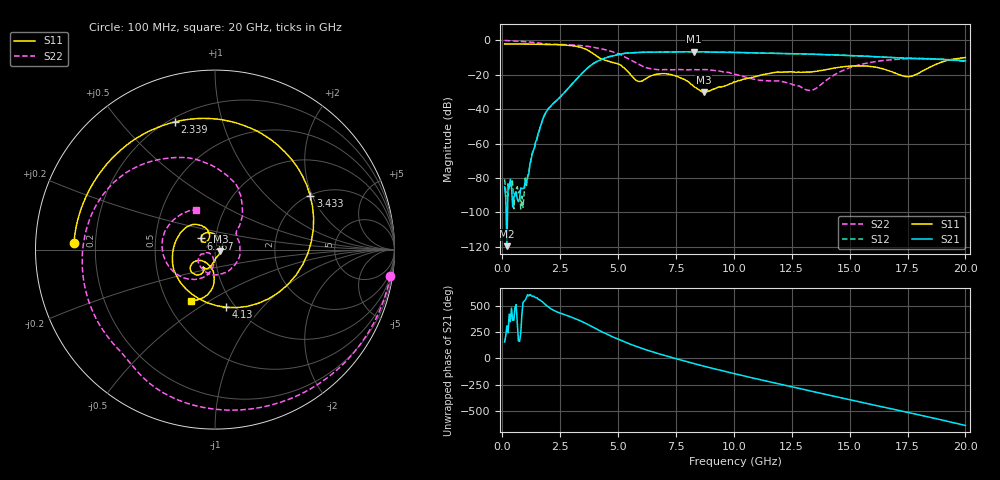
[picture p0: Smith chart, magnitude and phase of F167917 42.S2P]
!  2-Port S-parameters saved by WinCal
! VAR MeasName=S-Parameters (CALIBRATED_DATA) read from VNA (N5242A)
! VAR MeasDate=2016-11-22 9:01:51
! VAR NAME=F167917 42
! VAR FILENAME=F167917 42.S2P
! VAR DATE=2016-11-22 9:01:51
! VAR PHYS_PORTS=1,2
# Hz S DB R 50
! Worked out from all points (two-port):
!   401 points, 100 MHz to 20 GHz, reference 50 ohm
!   highest |S21| = -6.61 dB at 8.259 GHz (marker M1); lowest = -119.6 dB at 199.5 MHz (marker M2)
!   |S21| within 3 dB of the highest: 4.596 GHz to 16.25 GHz (11.66 GHz wide, 112 % of centre)
!   lowest |S11| = -30.1 dB at 8.707 GHz (marker M3), VSWR 1.06, Z = 53.1 - j0.995 ohm
!   |S11| at or under -10 dB: 4.166 GHz to end of sweep
!   |S22| runs from -29.1 to -0.1 dB; largest |S21 - S12| = 0.0059
!   S11 on the Smith chart (normalised r, x): 100 MHz: 0.12, +0.02; 2.339 GHz: 0.22, +0.71; 3.433 GHz: 2.03, +1.93; 4.13 GHz: 0.91, -0.65; 6.567 GHz: 0.85, +0.11; 20 GHz: 0.66, -0.42
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1e8  -2.09 177.3  -85.10 156.0  -80.76 154.0  -0.10 -8.7
1.995e8  -2.10 174.7  -119.60 -49.3  -90.77 -77.3  -0.16 -16.9
1.04525e9  -2.23 151.9  -82.88 -137.0  -84.39 -79.3  -0.87 -80.9
1.74175e9  -2.35 130.7  -46.18 179.4  -46.16 179.3  -1.95 -124.1
2.33875e9  -2.55 107.4  -35.04 86.1  -34.99 85.9  -2.33 -151.7
2.93575e9  -3.03 74.0  -26.60 37.7  -26.63 37.6  -2.65 -180.0
3.43325e9  -4.30 29.5  -19.34 -7.8  -19.36 -7.7  -3.10 156.1
4.12975e9  -9.70 -79.1  -12.03 -87.1  -11.99 -87.1  -4.57 121.9
4.5775e9  -12.11 -162.6  -9.67 -135.1  -9.63 -135.4  -5.95 99.8
5.22425e9  -15.66 123.7  -7.76 163.3  -7.75 163.0  -9.15 67.5
5.871e9  -23.83 127.1  -7.07 107.9  -7.07 107.8  -13.82 46.0
6.5675e9  -19.98 141.8  -6.90 57.2  -6.90 57.0  -16.77 34.8
6.7665e9  -19.51 134.3  -6.85 43.9  -6.86 43.7  -17.10 29.2
8.259e9  -26.73 37.5  -6.61 -48.1  -6.63 -48.0  -17.03 -62.3
8.70675e9  -30.13 -17.5  -6.73 -74.3  -6.74 -74.3  -16.98 -91.2
1.005e10  -24.09 -92.8  -7.05 -146.8  -7.05 -146.7  -19.76 -152.7
1.19405e10  -18.54 -117.2  -7.67 117.3  -7.62 117.1  -23.63 -160.2
1.338325e10  -18.34 -119.9  -8.08 45.5  -8.05 45.7  -28.98 -124.5
1.467675e10  -15.45 -123.3  -8.70 -17.7  -8.66 -17.8  -17.75 -102.9
1.67165e10  -17.73 -149.6  -9.89 -116.5  -9.93 -116.4  -11.37 -157.2
1.7612e10  -21.03 -117.0  -10.50 -159.0  -10.42 -159.1  -10.62 178.3
2e10  -10.04 -115.0  -11.92 80.8  -11.80 80.5  -12.27 115.2
